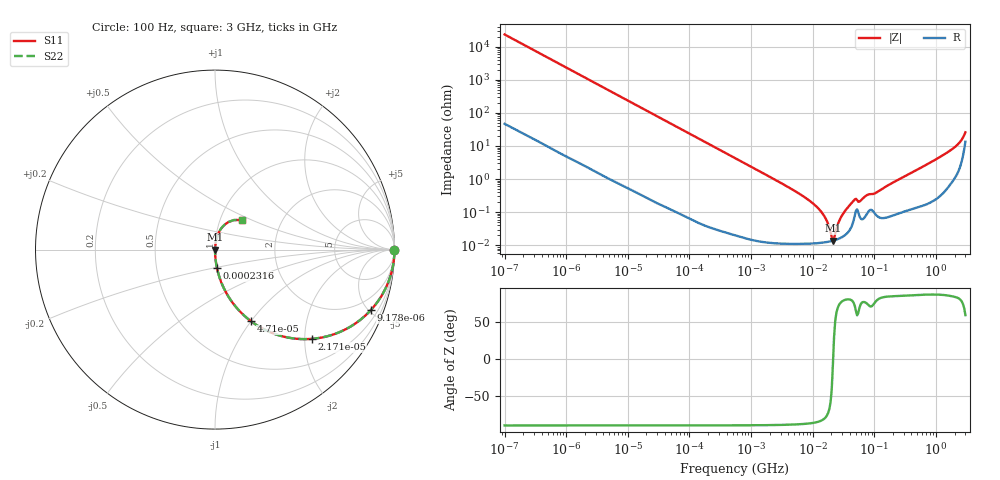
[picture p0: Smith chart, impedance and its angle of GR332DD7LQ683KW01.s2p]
!Murata Part Number: GR332DD7LQ683KW01
!These Parameters are Measured in Series Mode Connection
!Data Generated on Jan 08, 2026
!  o--ll--o
!Port1  Port2
!  o------o
!Operation Temp=25[degC], DC Bias Voltage=0[V]
!Freq. Start=100[Hz] Stop=3[GHz] 401[Steps]
# Hz S RI R 50
!Freq.(Hz) S11(Real) S11(Imag) S21(Real) S21(Imag) S12(Real) S12(Imag) S22(Real) S22(Imag)
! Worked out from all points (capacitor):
!   401 points, 100 Hz to 3 GHz, reference 50 ohm
!   read as one part in series: C = 68 nF near 109 Hz
!   lowest |Z| = 13.9 mohm at 21.25 MHz (marker M1)
!   series resonance near 21.43 MHz, so ESL is about 810 pH
!   S11 on the Smith chart (normalised r, x): 100 Hz: open; 9.178 kHz: 1.01, -5.13; 21.71 kHz: 1.01, -2.17; 47.1 kHz: 1.00, -1.00; 231.6 kHz: 1.00, -0.20; 3 GHz: 1.27, +0.44
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100  1 -0.00427  2.68e-05 0.00427  2.68e-05 0.00427  1 -0.00427
1788  0.9941 -0.0757  0.00592 0.0757  0.00592 0.0757  0.9941 -0.0757
9178  0.8675 -0.3379  0.1325 0.3379  0.1325 0.3379  0.8675 -0.3379
21707  0.541 -0.4972  0.459 0.4972  0.459 0.4972  0.541 -0.4972
31977  0.3526 -0.4766  0.6474 0.4766  0.6474 0.4766  0.3526 -0.4766
47105  0.2012 -0.3996  0.7988 0.3996  0.7988 0.3996  0.2012 -0.3996
89839  0.0652 -0.2456  0.9348 0.2456  0.9348 0.2456  0.0652 -0.2456
231582  0.0106 -0.101  0.9894 0.101  0.9894 0.101  0.0106 -0.101
547723  0.00206 -0.0431  0.9979 0.0431  0.9979 0.0431  0.00206 -0.0431
4141163  0.000141 -0.00552  0.9999 0.00552  0.9999 0.00552  0.000141 -0.00552
9794414  0.000117 -0.00192  0.9999 0.00192  0.9999 0.00192  0.000117 -0.00192
1.506283e7  0.000122 -0.000802  0.9999 0.000802  0.9999 0.000802  0.000122 -0.000802
2.12544e7  0.000138 -1.78e-05  0.9999 1.78e-05  0.9999 1.78e-05  0.000138 -1.78e-05
2.316512e7  0.000144 0.000177  0.9999 -0.000177  0.9999 -0.000177  0.000144 0.000177
2.635803e7  0.000158 0.000475  0.9998 -0.000475  0.9998 -0.000475  0.000158 0.000475
2.999103e7  0.000178 0.000788  0.9998 -0.000788  0.9998 -0.000788  0.000178 0.000788
4.612319e7  0.000573 0.00217  0.9994 -0.00217  0.9994 -0.00217  0.000573 0.00217
5.9714e7  0.000652 0.00212  0.9993 -0.00212  0.9993 -0.00212  0.000652 0.00212
1.751444e8  0.000776 0.0068  0.9992 -0.0068  0.9992 -0.0068  0.000776 0.0068
1.506733e9  0.00892 0.0618  0.9911 -0.0618  0.9911 -0.0618  0.00892 0.0618
2.219584e9  0.0253 0.1028  0.9747 -0.1028  0.9747 -0.1028  0.0253 0.1028
3e9  0.1504 0.1653  0.8496 -0.1653  0.8496 -0.1653  0.1504 0.1653
